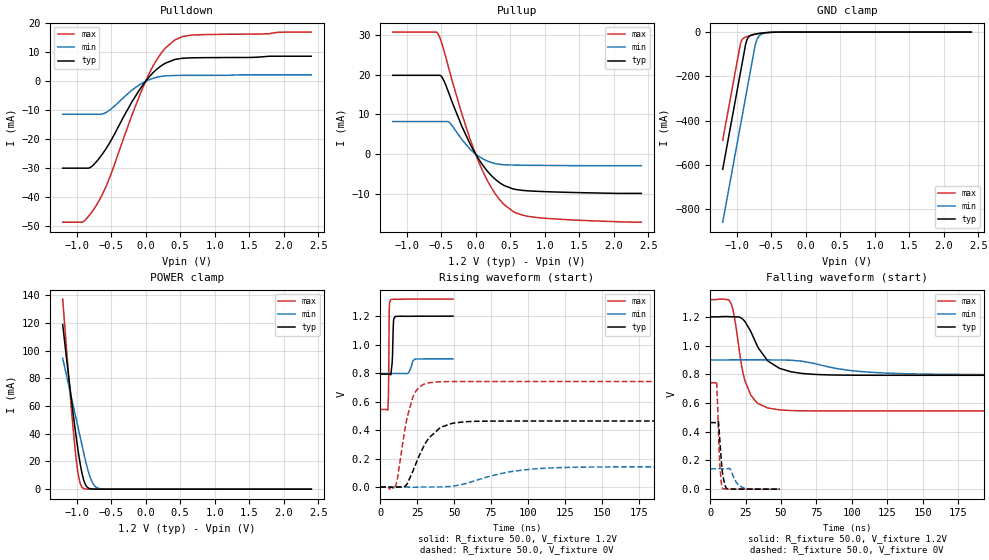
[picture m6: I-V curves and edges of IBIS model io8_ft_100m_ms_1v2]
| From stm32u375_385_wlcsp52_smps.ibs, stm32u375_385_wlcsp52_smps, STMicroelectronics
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[Model]   io8_ft_100m_ms_1v2
Model_type I/O
Polarity   Non-Inverting
Enable   Active-Low
| CAP_THRESHOLD on pad IOFT is "UDTCAPC" :
| Rising=30.0% of vddiom   Falling=70.0% of vddiom
| C_comp min and max val. don't necessarily correlate with the min and max pvt
| but are the smallest and greatest pad capacitance found.
| var   typ   min   max
C_comp   2.92097pF  2.86112pF  2.97372pF
|C_comp_pullup   1.65808pF  1.48843pF  1.79606pF
|C_comp_pulldown   1.26290pF  1.37269pF  1.17766pF
Vinl = 450.0mV
Vinh = 660.0mV
Vmeas = 600.0mV   | Reference voltage for timing measurements
Cref  = 50.0pF   | Timing specification test load capacitance value
Rref  = 1.0MOhm   | Timing specification test load resistance value
Vref  = 660.0mV   | Timing specification test load voltage
[Model Spec]
| TIME_THRESHOLD on pin ZIV11 is "CMOS" :
| Rising=50.0% of vdd   Falling=50.0% of vdd
Vinl 439.50000mV 331.50001mV 485.50000mV
Vinh 752.50000mV 552.50001mV 837.50000mV
| variable   typ   min   max
[Temperature Range] 25.0 130.0 -40.0
| variable   typ   min   max
[Voltage Range] 1.2V 900.0mV 1.32V
| variable   typ   min   max
[POWER Clamp Reference] 1.2V 900.0mV 1.32V
| variable   typ   min   max
[GND Clamp Reference] 0V 0V 0V
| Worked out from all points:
|   slope of the pulldown table from 0 to 0.18 V, typ, clamps not added: 40 ohm
|   slope of the pullup table from 0 to 0.18 V, typ, clamps not added: 40 ohm
|   GND clamp passes 1 mA (typ) near -0.50 V on its own axis
|   POWER clamp passes 1 mA (typ) near -0.83 V on its own axis
|   rising waveform, R_fixture 50.0, V_fixture 1.2V: 20-80 % time 717ps typ, 1.98ns min, 394ps max; typ from 0.793 V to 1.2 V
|   falling waveform, R_fixture 50.0, V_fixture 1.2V: 20-80 % time 16.2ns typ, 36.8ns min, 9.15ns max; typ from 1.2 V to 0.793 V
|   rising waveform, R_fixture 50.0, V_fixture 0V: 20-80 % time 14.4ns typ, 33.4ns min, 8.09ns max; typ from 0 V to 0.464 V
|   falling waveform, R_fixture 50.0, V_fixture 0V: 20-80 % time 2.43ns typ, 4.77ns min, 1.78ns max; typ from 0.464 V to 0 V
[POWER Clamp]
-1.2V     118.8mA    94.44mA    137.2mA
-1.09V    71.2mA     69.75mA    67.14mA
-1.02V    43.22mA    54.03mA    28.67mA
-990mV    32.26mA    47.3mA     15.78mA
-970mV    25.49mA    42.81mA    9.257mA
-940mV    16.45mA    36.08mA    3.257mA
-910mV    9.238mA    29.34mA    904.6uA
-860mV    2.387mA    18.53mA    87.46uA
-790mV    204.6uA    7.049mA    3.101uA
-730mV    21.91uA    2.041mA    176.4nA
-660mV    1.594uA    337.6uA    6.285nA
2.4V      0A         0A         0A
[GND Clamp]
-1.2V     -619mA     -857.5mA   -488.2mA
-950mV    -194mA     -432.5mA   -63.18mA
-930mV    -160mA     -398.5mA   -40.87mA
-870mV    -57.95mA   -296.5mA   -22.39mA
-840mV    -28.97mA   -245.5mA   -19.16mA
-800mV    -15.67mA   -177.5mA   -15.71mA
-730mV    -8.807mA   -59.89mA   -10.55mA
-700mV    -7.204mA   -30.66mA   -8.61mA
-660mV    -5.427mA   -13.83mA   -6.309mA
-580mV    -2.713mA   -4.125mA   -2.796mA
-380mV    -62.64uA   -240.2uA   -21.17uA
2.4V      836.4pA    121.5nA    348.6pA
| variable   typ   min   max
[Pullup Reference] 1.2V 900.0mV 1.32V
| variable   typ   min   max
[Pulldown Reference] 0V 0V 0V
[Pullup]
-1.2V     19.89mA    8.21mA     30.81mA
-550mV    19.89mA    8.21mA     30.54mA
-480mV    19.24mA    8.21mA     27.46mA
-380mV    15.06mA    7.993mA    21.15mA
-200mV    7.047mA    3.684mA    10.21mA
10mV      -293.8uA   -130.6uA   -448.5uA
210mV     -5.089mA   -2.027mA   -7.926mA
310mV     -6.737mA   -2.489mA   -10.64mA
420mV     -8mA       -2.709mA   -12.87mA
580mV     -8.947mA   -2.8mA     -14.83mA
790mV     -9.331mA   -2.845mA   -15.82mA
2.4V      -9.943mA   -2.948mA   -17.22mA
[Pulldown]
-1.2V     -29.93mA   -11.33mA   -48.55mA
-910mV    -29.93mA   -11.33mA   -48.48mA
-810mV    -29.8mA    -11.33mA   -46.03mA
-710mV    -27.65mA   -11.33mA   -42.6mA
-620mV    -24.89mA   -11.22mA   -38.69mA
-530mV    -21.58mA   -10.08mA   -33.79mA
-200mV    -7.157mA   -3.075mA   -11.82mA
40mV      1.18mA     424.7uA    2.081mA
230mV     5.395mA    1.701mA    9.799mA
420mV     7.512mA    2.016mA    14.19mA
670mV     8.097mA    2.046mA    15.93mA
2.4V      8.645mA    2.222mA    16.96mA
[Ramp]
dV/dt_r 278.13738mV/13.64144ns 85.17703mV/32.80269ns 444.65454mV/7.76094ns
dV/dt_f 244.21092mV/15.29887ns 61.56271mV/36.22157ns 465.10843mV/8.74957ns
R_load = 50.0
| Removed startup time: 0s 0s 0s  .
| Removed end time: 49.25ns.
[Rising Waveform]
R_fixture   = 50.0
V_fixture   = 1.2V
V_fixture_min = 900.0mV
V_fixture_max = 1.32V
0s        793mV      797.4mV    544.8mV
5.2ns     793mV      797.4mV    551.8mV
5.6ns     793.1mV    797.4mV    698mV
6.15ns    792.9mV    797.4mV    1.26V
7.05ns    788.7mV    797.4mV    1.316V
8.05ns    872.6mV    797.4mV    1.318V
9ns       1.168V     797.4mV    1.318V
10.05ns   1.197V     797.4mV    1.319V
23.15ns   1.199V     896.7mV    1.32V
49.25ns   1.2V       899.7mV    1.32V
| Removed startup time: 0s 0s 0s  .
| Removed end time: 399.25ns.
[Falling Waveform]
R_fixture   = 50.0
V_fixture   = 1.2V
V_fixture_min = 900.0mV
V_fixture_max = 1.32V
0s        1.2V       900mV      1.32V
14.3ns    1.201V     900.5mV    1.299V
16.75ns   1.2V       900.6mV    1.214V
24.45ns   1.168V     900.4mV    755.9mV
32.6ns    1.011V     900.4mV    606mV
40.75ns   892mV      900.1mV    565.2mV
57.05ns   817.4mV    898mV      547.4mV
81.5ns    796.3mV    856.2mV    544.9mV
146.7ns   793mV      802.2mV    544.8mV
399.3ns   793mV      797.4mV    544.8mV
| Removed startup time: 0s 0s 0s  .
| Removed end time: 399.2ns.
[Rising Waveform]
R_fixture   = 50.0
V_fixture   = 0V
V_fixture_min = 0V
V_fixture_max = 0V
0s        4.598nV    136nV      3.245nV
10.3ns    -1.301mV   544.5nV    7.354mV
11.85ns   -502.3uV   67.15nV    73.96mV
17.6ns    13.27mV    -30.2uV    456.8mV
22.05ns   109.7mV    -1.923mV   631.7mV
32.6ns    339.3mV    -68.59uV   731.5mV
40.75ns   418.6mV    97.63uV    739.4mV
60.9ns    460.2mV    33.8mV     741mV
122.2ns   463.5mV    136.4mV    741.1mV
399.2ns   463.6mV    142mV      741.1mV
| Removed startup time: 0s 0s 0s  .
| Removed end time: 49.25ns.
[Falling Waveform]
R_fixture   = 50.0
V_fixture   = 0V
V_fixture_min = 0V
V_fixture_max = 0V
0s        463.6mV    142mV      741.1mV
4.45ns    463.6mV    142mV      747.1mV
5.75ns    468mV      142mV      409.7mV
6.6ns     361mV      142mV      192.7mV
7.75ns    205mV      142mV      48.87mV
8.55ns    119.7mV    142mV      6.054mV
10.05ns   41.58mV    142mV      1.881mV
12.05ns   1.984mV    141.8mV    1.062mV
24.15ns   427uV      6.311mV    179.3uV
49.25ns   49.3uV     88uV       6.883uV
